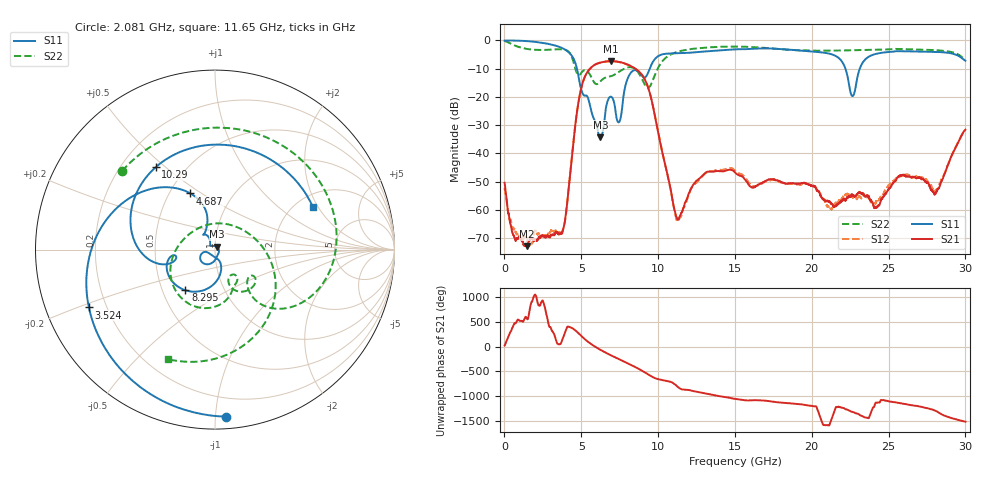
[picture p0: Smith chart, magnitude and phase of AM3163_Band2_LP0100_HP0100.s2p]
!Agilent Technologies,E8364B,MY43040894,A.07.50.67
!Agilent E8364B: A.07.50.67
!Date: Thursday, August 20, 2020 11:12:21
!Correction: S11(Full 2 Port(1,2))
!S21(Full 2 Port(1,2))
!S12(Full 2 Port(1,2))
!S22(Full 2 Port(1,2))
!S2P File: Measurements: S11, S21, S12, S22:
# Hz S  dB  R 50
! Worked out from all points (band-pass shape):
!   3201 points, 10 MHz to 30 GHz, reference 50 ohm
!   highest |S21| = -7.38 dB at 6.945 GHz (marker M1); lowest = -72.8 dB at 1.472 GHz (marker M2)
!   |S21| within 3 dB of the highest: 5.511 GHz to 8.609 GHz (3.098 GHz wide, 43.9 % of centre)
!   lowest |S11| = -34.3 dB at 6.242 GHz (marker M3), VSWR 1.04, Z = 51.1 + j1.6 ohm
!   |S11| at or under -10 dB: 4.718 GHz to 9.458 GHz (4.74 GHz wide, 66.9 % of centre); 22.19 GHz to 23.13 GHz (934.7 MHz wide, 4.13 % of centre)
!   |S22| runs from -16.8 to -0.3 dB; largest |S21 - S12| = 0.0053
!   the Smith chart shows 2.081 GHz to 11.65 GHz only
!   S11 on the Smith chart (normalised r, x): 2.081 GHz: 0.07, -1.07; 3.524 GHz: 0.13, -0.21; 4.687 GHz: 0.63, +0.45; 8.295 GHz: 0.65, -0.32; 10.29 GHz: 0.34, +0.46; 11.65 GHz: 2.48, +1.80
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1e7  -0.09 -2.7  -50.36 23.0  -52.18 -124.4  -0.27 -10.8
6.098e8  -0.08 -24.7  -69.20 88.7  -66.82 -90.5  -1.69 -87.4
1.472012e9  -0.29 -60.3  -72.77 -157.4  -69.85 -171.5  -3.06 -173.6
2.081184e9  -0.60 -86.2  -70.90 -84.2  -67.87 -81.0  -3.38 139.8
3.524453e9  -2.24 -155.3  -68.50 48.2  -67.88 91.7  -3.16 39.4
4.686566e9  -9.32 113.7  -26.69 -50.2  -26.72 -50.6  -11.26 -48.4
5.014581e9  -17.76 111.6  -16.50 -146.9  -16.52 -147.1  -11.41 -34.7
6.242297e9  -34.28 53.8  -7.87 -64.0  -7.89 -64.1  -14.53 -51.0
6.945188e9  -19.95 -139.9  -7.38 -177.5  -7.39 -177.6  -12.67 -63.8
7.460641e9  -28.90 -116.3  -7.65 105.2  -7.68 105.0  -11.13 -74.4
8.294738e9  -11.05 -126.0  -9.30 -18.9  -9.32 -18.7  -9.56 -119.6
1.000979e10  -5.58 150.5  -32.83 61.5  -32.72 60.2  -9.65 -14.9
1.029095e10  -4.95 125.7  -40.07 43.9  -40.01 41.5  -7.31 -39.9
1.164987e10  -4.50 23.2  -59.26 -146.6  -59.29 -144.8  -3.54 -113.4
1.333681e10  -3.81 -72.0  -46.40 114.5  -46.30 119.0  -2.49 -172.5
1.5005e10  -3.20 -143.1  -46.73 21.7  -46.04 24.2  -2.22 131.6
1.771347e10  -2.96 94.4  -49.51 -43.8  -49.70 -45.0  -3.03 30.5
2.000958e10  -3.97 -27.6  -51.49 -120.5  -51.27 -118.0  -3.66 -50.2
2.265245e10  -19.73 -108.0  -54.57 119.0  -55.44 121.6  -3.52 -124.6
2.500479e10  -4.13 -151.1  -52.52 -25.5  -51.19 -19.0  -3.20 178.0
2.806939e10  -4.10 113.5  -54.00 138.6  -52.92 139.3  -3.46 96.8
3e10  -7.23 41.7  -31.62 -78.1  -31.78 -77.9  -6.90 37.4
